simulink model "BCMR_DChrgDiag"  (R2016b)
settings: Solver=FixedStepDiscrete  StartTime=0.0  StopTime=10  FixedStep=0.01  RelTol=1e-3  EnableMultiTasking=on
undefined symbols (not defined in the file or in its folder): BCMR_bDChrgStopCActiveSw_C, BCMR_cntDChrgTCnntMax_C, BCMR_cntIsoFltTrigger_CW, BCMR_EVCCDiagccSw_C, BCMR_EVCCDiagSw_C, BCMR_G1E0PlatformSwDiag_C, BCMR_H1U0PlatformSwDiag_C, BCMR_iDcChrgDiffOvrCurr_C, BCMR_iDcChrgLowTempDiffOvrCurrMody_C, BCMR_iDcChrgLowTempOvrCurrCutOff_C, BCMR_iDcChrgLowTempOvrCurrHeal_C, BCMR_iDcChrgOvrCurr_C, BCMR_iDcChrgOvrVolt_C, BCMR_iDChrgCurrDiagLmt_C, BCMR_iDChrgCutOffVoltOvrCurrDet_C, BCMR_iDChrgCutOffVoltOvrCurrHeal_C, BCMR_kWaveFltFactor_C, BCMR_stCCSTimeout_C, BCMR_stCHMTimeout_C, BCMR_stCMLTimeout_C, BCMR_stCRMAATimeout_C, BCMR_stCROAATimeout_C, BCMR_stCROTimeout_C, BCMR_stCSDTimeout1_C, BCMR_stCSDTimeout2_C, BCMR_stCSTTimeout_C, BCMR_stCurrDwnTimeout_C, BCMR_stHvOnTimeout_C, BCMR_stNoTimeout_C, BCMR_stParaMish_C, BCMR_tBattLowTempDiagTempThrd_C, BCMR_tDcChrgIntfTempDiffLmt_C, BCMR_tDcChrgIntfTempLmt_C, BCMR_tiDChrgDetDiagDebs_C, BCMR_tiDChrgDetSec_C, BCMR_tiDChrgDiagBase_C, BCMR_tiDChrgHealDiagDebs_C, BCMR_tiDChrgIntfTempDwnLmt_C, BCMR_tiDChrgLowTOvrCurrDet_C, BCMR_tiDChrgLowTOvrCurrHeal_C, BCMR_tiDChrgMishCurrDetDiagDebs_C, BCMR_tiDChrgOvrCellVolt_C, BCMR_tiDChrgOvrSafeCellVoltDet_C, BCMR_tiDChrgVoltFltDetDebs_C, BCMR_tiDChrgVoltFltHealDebs_C, BCMR_uCC2ChkDiffDet_C, BCMR_uCC2ChkDiffHeal_C, BCMR_uCC2VoltHighDet_C, BCMR_uCC2VoltHighHeal_C, BCMR_uCC2VoltLowDet_C, BCMR_uCC2VoltLowHeal_C, BCMR_uDChrgHighTempDet_C, BCMR_uDChrgHighTempHeal_C, BCMR_uDChrgLowTempDet_C, BCMR_uDChrgLowTempHeal_C, BCMR_uDChrgOvrCellVoltDet_C, BCMR_uDChrgOvrCellVoltHeal_C, BCMR_uDChrgOvrSafeCellVoltDet_C, BCMR_uDChrgOvrSafeCellVoltHeal_C, bin2dec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
libraries: simulink x291
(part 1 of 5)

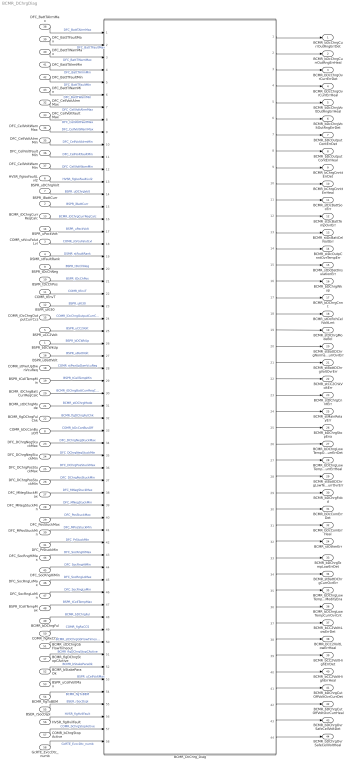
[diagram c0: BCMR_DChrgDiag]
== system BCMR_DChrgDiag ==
  BSPR_bDCWkUp : Inport
  BSPR_iBattCurr : Inport  Port=2
  COMR_stVcuFalutLvl : Inport  Port=3
  DSMR_stFaultRank : Inport  Port=4
  BSPR_uCC2Volt : Inport  Port=5
  HVSR_flgIsoFaultLvl2 : Inport  Port=6
  BSPR_uDChrgVolt : Inport  Port=7
  COMR_bDcCanBusOff : Inport  Port=8
  BSPR_tDcChNeg : Inport  Port=9
  BSPR_tDcChPos : Inport  Port=10
  COMR_tEnvT : Inport  Port=11
  BSPR_uKl30 : Inport  Port=12
  BCMR_iDChrgCurrReqCalc : Inport  Port=13
  BSPR_uPackVolt : Inport  Port=14
  COMR_iDcChrgOutputCurrCcs : Inport  Port=15
  BSPR_uBattVolt : Inport  Port=16
  BCMR_flgDChrgStopCActive : Inport  Port=17
  COMR_stPwrUpDwnVcuReq : Inport  Port=18
  BSPR_tCellTempMin : Inport  Port=19
  BCMR_iDChrgBattCurrReqCalc : Inport  Port=20
  BCMR_stDChrgMode : Inport  Port=21
  BCMR_flgDChrgFulChk : Inport  Port=22
  DFC_DChrgNegStuckMax : Inport  Port=23
  DFC_DChrgNegStuckMin : Inport  Port=24
  DFC_DChrgPosStuckMax : Inport  Port=25
  DFC_DChrgPosStuckMin : Inport  Port=26
  DFC_MNegStuckMax : Inport  Port=27
  DFC_MNegStuckMin : Inport  Port=28
  DFC_PosStuckMax : Inport  Port=29
  DFC_MPosStuckMin : Inport  Port=30
  DFC_PrStuckMin : Inport  Port=31
  DFC_CellVoltAlrmMax : Inport  Port=32
  DFC_CellVoltFaultMax : Inport  Port=33
  DFC_CellVoltWarnMax : Inport  Port=34
  DFC_CellVoltAlrmMin : Inport  Port=35
  DFC_CellVoltFaultMin : Inport  Port=36
  DFC_CellVoltWarnMin : Inport  Port=37
  DFC_BattTAlrmMax : Inport  Port=38
  DFC_BattTFaultMax : Inport  Port=39
  "DFC_BattTWarnMax " : Inport  Port=40
  DFC_BattTAlrmMin : Inport  Port=41
  DFC_BattTFaultMin : Inport  Port=42
  DFC_BattTWarnMin : Inport  Port=43
  DFC_SocRngHiMax : Inport  Port=44
  DFC_SocRngHiMin : Inport  Port=45
  DFC_SocRngLoMax : Inport  Port=46
  DFC_SocRngLoMin : Inport  Port=47
  BSPR_tCellTempMax : Inport  Port=48
  BCMR_bDChrgFul : Inport  Port=49
  COMR_flgRxCCS : Inport  Port=50
  BCMR_stDChrgGbFlowTimeout : Inport  Port=51
  BCMR_bStakeParaOk : Inport  Port=52
  BSPR_uCellVoltMax : Inport  Port=53
  BCMR_flgTxBEM : Inport  Port=54
  BSER_rSocDspl : Inport  Port=55
  HVSR_flgHvilFault : Inport  Port=56
  COMR_bChrgStopActive : Inport  Port=57
  GcRTE_EvccDtc_numb : Inport  Port=58
  BCMR_DcChrg_Diag : Subsystem
  BCMR_bDcChrgCurrOutRngErrDet : Outport  InitialOutput=[0]
  BCMR_bDcChrgCurrOutRngErrHeal : Outport  Port=2  InitialOutput=[0]
  BCMR_bDcChrgOvrCurrErrDet : Outport  Port=3  InitialOutput=[0]
  BCMR_bDcChrgOvrCurrErrHeal : Outport  Port=4  InitialOutput=[0]
  BCMR_bDcChrgVoltOutRngErrHeal : Outport  Port=5  InitialOutput=[0]
  BCMR_bDcChrgVoltOutRngErrDet : Outport  Port=6  InitialOutput=[0]
  BCMR_bDcOutputContErrDet : Outport  Port=7  InitialOutput=[0]
  BCMR_bDcOutputContErrHeal : Outport  Port=8  InitialOutput=[0]
  BCMR_bChrgCnnttErrDet : Outport  Port=9  InitialOutput=[0]
  BCMR_bChrgCnnttErrHeal : Outport  Port=10  InitialOutput=[0]
  BCMR_stDcBattSocErr : Outport  Port=11
  BCMR_stDcBattTempOvrErr : Outport  Port=12
  BCMR_stDcBattCellVoltErr : Outport  Port=13
  BCMR_stDcOutpCnntOvrTempErr : Outport  Port=14  OutDataTypeStr=uint8
  BCMR_stDcBattInsulationErr : Outport  Port=15
  BCMR_bDChrgWkup : Outport  Port=16
  BCMR_bDChrgCnnt : Outport  Port=17
  BCMR_stDcRchCellVoltLmt : Outport  Port=18  OutDataTypeStr=uint8
  BCMR_stDChrgModeBcl : Outport  Port=19  InitialOutput=[0]
  BCMR_stBattDChrgNormalTempCurrOvrErr : Outport  Port=20
  BCMR_stBattDChrgVoltOvrErr : Outport  Port=21
  BCMR_stCC2ChkVoltErr : Outport  Port=22
  BCMR_stDChrgCnntErr : Outport  Port=23  InitialOutput=[0]
  BCMR_stOtherErr : Outport  Port=24
  BCMR_stMainRelayErr : Outport  Port=25
  BCMR_bDChrgStopEna : Outport  Port=26
  BCMR_bDChrgLowTempOvrCurrErrDet : Outport  Port=27
  BCMR_bDChrgLowTempOvrCurrErrHeal : Outport  Port=28
  BCMR_stBattDChrgLowTempCurrOvrErr : Outport  Port=29
  BCMR_bDChrgFobd : Outport  Port=30
  BCMR_bDcComErrDet : Outport  Port=31
  BCMR_bDcComErrHeal : Outport  Port=32
  BCMR_bDChrgTempLowErrDet : Outport  Port=33
  BCMR_stBattDChrgCurrOvrErr : Outport  Port=34  InitialOutput=[0]
  BCMR_bDChrgLowTempCurrModifyEna : Outport  Port=35
  BCMR_bDChrgLowTempCurrOvrCnt : Outport  Port=36  OutputWhenDisabled=reset  InitialOutput=[0]
  BCMR_bCC2VolttLowErrDet : Outport  Port=37  InitialOutput=[0]
  BCMR_bCC2VoltLowErrHeal : Outport  Port=38  InitialOutput=[0]
  BCMR_bCC2VoltHighErrDet : Outport  Port=39  InitialOutput=[0]
  BCMR_bCC2VoltHighErrHeal : Outport  Port=40  InitialOutput=[0]
  BCMR_bDChrgCutOffVoltOvrCurrDet : Outport  Port=41
  BCMR_bDChrgCutOffVoltOvrCurrHeal : Outport  Port=42
  BCMR_bDChrgOvrSafeCellVoltDet : Outport  Port=43
  BCMR_bDChrgOvrSafeCellVoltHeal : Outport  Port=44
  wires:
  HVSR_flgIsoFaultLvl2/1 -> BCMR_DcChrg_Diag/13(HVSR_flgIsoFaultLvl2)  "HVSR_flgIsoFaultLvl2"
  BSPR_uDChrgVolt/1 -> BCMR_DcChrg_Diag/14(BSPR_uDChrgVolt)  "BSPR_uDChrgVolt"
  BSPR_iBattCurr/1 -> BCMR_DcChrg_Diag/15(BSPR_iBattCurr)  "BSPR_iBattCurr"
  COMR_bDcCanBusOff/1 -> BCMR_DcChrg_Diag/33(COMR_bDcCanBusOff)  "COMR_bDcCanBusOff"
  COMR_stVcuFalutLvl/1 -> BCMR_DcChrg_Diag/18(COMR_stVcuFalutLvl)  "COMR_stVcuFalutLvl"
  DSMR_stFaultRank/1 -> BCMR_DcChrg_Diag/19(DSMR_stFaultRank)  "DSMR_stFaultRank"
  BSPR_tDcChNeg/1 -> BCMR_DcChrg_Diag/20(BSPR_tDcChNeg)  "BSPR_tDcChNeg"
  BSPR_tDcChPos/1 -> BCMR_DcChrg_Diag/21(BSPR_tDcChPos)  "BSPR_tDcChPos"
  BSPR_uKl30/1 -> BCMR_DcChrg_Diag/23(BSPR_uKl30)  "BSPR_uKl30"
  COMR_tEnvT/1 -> BCMR_DcChrg_Diag/22(COMR_tEnvT)  "COMR_tEnvT"
  BSPR_bDCWkUp/1 -> BCMR_DcChrg_Diag/26(BSPR_bDCWkUp)  "BSPR_bDCWkUp"
  BSPR_uCC2Volt/1 -> BCMR_DcChrg_Diag/25(BSPR_uCC2Volt)  "BSPR_uCC2Volt"
  BCMR_iDChrgCurrReqCalc/1 -> BCMR_DcChrg_Diag/16(BCMR_iDChrgCurrReqCalc)  "BCMR_iDChrgCurrReqCalc"
  BSPR_uPackVolt/1 -> BCMR_DcChrg_Diag/17(BSPR_uPackVolt)  "BSPR_uPackVolt"
  COMR_iDcChrgOutputCurrCcs/1 -> BCMR_DcChrg_Diag/24(COMR_iDcChrgOutputCurrCcs)  "COMR_iDcChrgOutputCurrCcs"
  BSPR_uBattVolt/1 -> BCMR_DcChrg_Diag/27(BSPR_uBattVolt)  "BSPR_uBattVolt"
  BCMR_flgDChrgStopCActive/1 -> BCMR_DcChrg_Diag/51(BCMR_flgDChrgStopCActive)  "BCMR_flgDChrgStopCActive"
  BCMR_DcChrg_Diag/13(BCMR_stDcBattCellVoltErr) -> BCMR_stDcBattCellVoltErr/1
  BCMR_DcChrg_Diag/22(BCMR_stCC2ChkVoltErr) -> BCMR_stCC2ChkVoltErr/1
  BCMR_DcChrg_Diag/1(BCMR_bDcChrgCurrOutRngErrDet) -> BCMR_bDcChrgCurrOutRngErrDet/1
  BCMR_DcChrg_Diag/2(BCMR_bDcChrgCurrOutRngErrHeal) -> BCMR_bDcChrgCurrOutRngErrHeal/1
  BCMR_DcChrg_Diag/3(BCMR_bDcChrgOvrCurrErrDet) -> BCMR_bDcChrgOvrCurrErrDet/1
  BCMR_DcChrg_Diag/4(BCMR_bDcChrgOvrCurrErrHeal) -> BCMR_bDcChrgOvrCurrErrHeal/1
  BCMR_DcChrg_Diag/6(BCMR_bDcChrgVoltOutRngErrDet) -> BCMR_bDcChrgVoltOutRngErrDet/1
  BCMR_DcChrg_Diag/5(BCMR_bDcChrgVoltOutRngErrHeal) -> BCMR_bDcChrgVoltOutRngErrHeal/1
  BCMR_DcChrg_Diag/7(BCMR_bDcOutputContErrDet) -> BCMR_bDcOutputContErrDet/1
  BCMR_DcChrg_Diag/8(BCMR_bDcOutputContErrHeal) -> BCMR_bDcOutputContErrHeal/1
  BCMR_DcChrg_Diag/9(BCMR_bChrgCnnttErrDet) -> BCMR_bChrgCnnttErrDet/1
  BCMR_DcChrg_Diag/10(BCMR_bChrgCnnttErrHeal) -> BCMR_bChrgCnnttErrHeal/1
  BCMR_DcChrg_Diag/11(BCMR_stDcBattSocErr) -> BCMR_stDcBattSocErr/1
  BCMR_DcChrg_Diag/12(BCMR_stDcBattTempOvrErr) -> BCMR_stDcBattTempOvrErr/1
  BCMR_DcChrg_Diag/16(BCMR_bDChrgWkup) -> BCMR_bDChrgWkup/1
  BCMR_DcChrg_Diag/17(BCMR_bDChrgCnnt) -> BCMR_bDChrgCnnt/1
  BCMR_DcChrg_Diag/18(BCMR_stDcRchCellVoltLmt) -> BCMR_stDcRchCellVoltLmt/1
  BCMR_DcChrg_Diag/15(BCMR_stDcBattInsulationErr) -> BCMR_stDcBattInsulationErr/1
  BCMR_DcChrg_Diag/14(BCMR_stDcOutpCnntOvrTempErr) -> BCMR_stDcOutpCnntOvrTempErr/1
  BCMR_DcChrg_Diag/19(BCMR_stDChrgModeBcl) -> BCMR_stDChrgModeBcl/1
  BCMR_DcChrg_Diag/20(BCMR_stBattNormalTempDChrgCurrOvrErr) -> BCMR_stBattDChrgNormalTempCurrOvrErr/1
  BCMR_DcChrg_Diag/23(BCMR_stDChrgCnntErr) -> BCMR_stDChrgCnntErr/1
  BCMR_DcChrg_Diag/21(BCMR_stBattDChrgVoltOvrErr) -> BCMR_stBattDChrgVoltOvrErr/1
  BCMR_DcChrg_Diag/32(BCMR_stOtherErr) -> BCMR_stOtherErr/1
  BCMR_DcChrg_Diag/24(BCMR_stMainRelayErr) -> BCMR_stMainRelayErr/1
  COMR_stPwrUpDwnVcuReq/1 -> BCMR_DcChrg_Diag/28(COMR_stPwrUpDwnVcuReq)  "COMR_stPwrUpDwnVcuReq"
  BCMR_DcChrg_Diag/25(BCMR_bDChrgStopEna) -> BCMR_bDChrgStopEna/1
  BSPR_tCellTempMin/1 -> BCMR_DcChrg_Diag/29(BSPR_tBattTempMin)  "BSPR_tCellTempMin"
  BCMR_iDChrgBattCurrReqCalc/1 -> BCMR_DcChrg_Diag/30(BCMR_iDChrgBattCurrReqCalc)  "BCMR_iDChrgBattCurrReqCalc"
  BCMR_DcChrg_Diag/26(BCMR_bDChrgLowTempOvrCurrErrDet) -> BCMR_bDChrgLowTempOvrCurrErrDet/1
  BCMR_DcChrg_Diag/27(BCMR_bDChrgLowTempOvrCurrErrHeal) -> BCMR_bDChrgLowTempOvrCurrErrHeal/1
  BCMR_DcChrg_Diag/28(BCMR_stBattDChrgLowTempCurrOvrErr) -> BCMR_stBattDChrgLowTempCurrOvrErr/1
  BCMR_DcChrg_Diag/29(BCMR_bDChrgFobd) -> BCMR_bDChrgFobd/1
  BCMR_stDChrgMode/1 -> BCMR_DcChrg_Diag/31(BCMR_stDChrgMode)  "BCMR_stDChrgMode"
  BCMR_flgDChrgFulChk/1 -> BCMR_DcChrg_Diag/32(BCMR_flgDChrgFulChk)  "BCMR_flgDChrgFulChk"
  BCMR_DcChrg_Diag/31(BCMR_bDcComErrHeal) -> BCMR_bDcComErrHeal/1
  BCMR_DcChrg_Diag/30(BCMR_bDcComErrDet) -> BCMR_bDcComErrDet/1
  DFC_DChrgNegStuckMax/1 -> BCMR_DcChrg_Diag/34(DFC_DChrgNegStuckMax)  "DFC_DChrgNegStuckMax"
  DFC_DChrgNegStuckMin/1 -> BCMR_DcChrg_Diag/35(DFC_DChrgNegStuckMin)  "DFC_DChrgNegStuckMin"
  DFC_DChrgPosStuckMax/1 -> BCMR_DcChrg_Diag/36(DFC_DChrgPosStuckMax)  "DFC_DChrgPosStuckMax"
  DFC_DChrgPosStuckMin/1 -> BCMR_DcChrg_Diag/37(DFC_DChrgPosStuckMin)  "DFC_DChrgPosStuckMin"
  DFC_MNegStuckMax/1 -> BCMR_DcChrg_Diag/38(DFC_MNegStuckMax)  "DFC_MNegStuckMax"
  DFC_MNegStuckMin/1 -> BCMR_DcChrg_Diag/39(DFC_MNegStuckMin)  "DFC_MNegStuckMin"
  DFC_PosStuckMax/1 -> BCMR_DcChrg_Diag/40(DFC_PosStuckMax)  "DFC_PosStuckMax"
  DFC_MPosStuckMin/1 -> BCMR_DcChrg_Diag/41(DFC_MPosStuckMin)  "DFC_MPosStuckMin"
  DFC_PrStuckMin/1 -> BCMR_DcChrg_Diag/42(DFC_PrStuckMin)  "DFC_PrStuckMin"
  DFC_CellVoltAlrmMax/1 -> BCMR_DcChrg_Diag/7(DFC_CellVoltAlrmMax)  "DFC_CellVoltAlrmMax"
  DFC_CellVoltFaultMin/1 -> BCMR_DcChrg_Diag/11(DFC_CellVoltFaultMin)  "DFC_CellVoltFaultMin"
  DFC_CellVoltFaultMax/1 -> BCMR_DcChrg_Diag/8(DFC_CellVoltFaultMax)  "DFC_CellVoltFaultMax"
  DFC_CellVoltWarnMax/1 -> BCMR_DcChrg_Diag/9(DFC_CellVoltWarnMax)  "DFC_CellVoltWarnMax"
  DFC_CellVoltAlrmMin/1 -> BCMR_DcChrg_Diag/10(DFC_CellVoltAlrmMin)  "DFC_CellVoltAlrmMin"
  DFC_CellVoltWarnMin/1 -> BCMR_DcChrg_Diag/12(DFC_CellVoltWarnMin)  "DFC_CellVoltWarnMin"
  DFC_BattTAlrmMax/1 -> BCMR_DcChrg_Diag/1(DFC_BattTAlrmMax)  "DFC_BattTAlrmMax"
  DFC_BattTFaultMax/1 -> BCMR_DcChrg_Diag/2(DFC_BattTFaultMax)  "DFC_BattTFaultMax"
  "DFC_BattTWarnMax "/1 -> BCMR_DcChrg_Diag/3("DFC_BattTWarnMax ")  "DFC_BattTWarnMax"
  DFC_BattTAlrmMin/1 -> BCMR_DcChrg_Diag/4(DFC_BattTAlrmMin)  "DFC_BattTAlrmMin"
  DFC_BattTFaultMin/1 -> BCMR_DcChrg_Diag/5(DFC_BattTFaultMin)  "DFC_BattTFaultMin"
  DFC_BattTWarnMin/1 -> BCMR_DcChrg_Diag/6(DFC_BattTWarnMin)  "DFC_BattTWarnMin"
  DFC_SocRngHiMax/1 -> BCMR_DcChrg_Diag/43(DFC_SocRngHiMax)  "DFC_SocRngHiMax"
  DFC_SocRngHiMin/1 -> BCMR_DcChrg_Diag/44(DFC_SocRngHiMin)  "DFC_SocRngHiMin"
  DFC_SocRngLoMax/1 -> BCMR_DcChrg_Diag/45(DFC_SocRngLoMax)  "DFC_SocRngLoMax"
  DFC_SocRngLoMin/1 -> BCMR_DcChrg_Diag/46(DFC_SocRngLoMin)  "DFC_SocRngLoMin"
  BCMR_DcChrg_Diag/33(BCMR_bDChrgTempLowErrDet) -> BCMR_bDChrgTempLowErrDet/1
  BSPR_tCellTempMax/1 -> BCMR_DcChrg_Diag/47(BSPR_tBattTempMax)  "BSPR_tCellTempMax"
  BCMR_DcChrg_Diag/34(BCMR_stBattDChrgCurrOvrErr) -> BCMR_stBattDChrgCurrOvrErr/1
  BCMR_bDChrgFul/1 -> BCMR_DcChrg_Diag/48(BCMR_bDChrgFul)  "BCMR_bDChrgFul"
  COMR_flgRxCCS/1 -> BCMR_DcChrg_Diag/49(COMR_flgRxCCS)  "COMR_flgRxCCS"
  BCMR_DcChrg_Diag/35(BCMR_bDChrgLowTempCurrModifyEna) -> BCMR_bDChrgLowTempCurrModifyEna/1
  BCMR_DcChrg_Diag/36(BCMR_bDChrgLowTempCurrOvrCnt) -> BCMR_bDChrgLowTempCurrOvrCnt/1
  BCMR_stDChrgGbFlowTimeout/1 -> BCMR_DcChrg_Diag/50(BCMR_stDChrgGbFlowTimeout)  "BCMR_stDChrgGbFlowTimeout"
  BCMR_bStakeParaOk/1 -> BCMR_DcChrg_Diag/52(BCMR_bStakeParaOk)  "BCMR_bStakeParaOk"
  BCMR_DcChrg_Diag/37(BCMR_bCC2VolttLowErrDet) -> BCMR_bCC2VolttLowErrDet/1
  BCMR_DcChrg_Diag/40(BCMR_bCC2VoltHighErrHeal) -> BCMR_bCC2VoltHighErrHeal/1
  BCMR_DcChrg_Diag/39(BCMR_bCC2VoltHighErrDet) -> BCMR_bCC2VoltHighErrDet/1
  BCMR_DcChrg_Diag/38(BCMR_bCC2VoltLowErrHeal) -> BCMR_bCC2VoltLowErrHeal/1
  BCMR_DcChrg_Diag/41(BCMR_bDChrgCutOffVoltOvrCurrDet) -> BCMR_bDChrgCutOffVoltOvrCurrDet/1
  BCMR_DcChrg_Diag/42(BCMR_bDChrgCutOffVoltOvrCurrHeal) -> BCMR_bDChrgCutOffVoltOvrCurrHeal/1
  BSPR_uCellVoltMax/1 -> BCMR_DcChrg_Diag/53(BSPR_uCellVoltMax)  "BSPR_uCellVoltMax"
  BCMR_flgTxBEM/1 -> BCMR_DcChrg_Diag/54(BCMR_flgTxBEM)  "BCMR_flgTxBEM"
  BSER_rSocDspl/1 -> BCMR_DcChrg_Diag/55(BSER_rSocDspl)  "BSER_rSocDspl"
  HVSR_flgHvilFault/1 -> BCMR_DcChrg_Diag/56(HVSR_flgHvilFault)  "HVSR_flgHvilFault"
  BCMR_DcChrg_Diag/43(BCMR_bDChrgOvrSafeCellVoltDet) -> BCMR_bDChrgOvrSafeCellVoltDet/1
  BCMR_DcChrg_Diag/44(BCMR_bDChrgOvrSafeCellVoltHeal) -> BCMR_bDChrgOvrSafeCellVoltHeal/1
  COMR_bChrgStopActive/1 -> BCMR_DcChrg_Diag/57(COMR_bChrgStopActive)  "COMR_bChrgStopActive"
  GcRTE_EvccDtc_numb/1 -> BCMR_DcChrg_Diag/58(GcRTE_EvccDtc_numb)  "GcRTE_EvccDtc_numb"

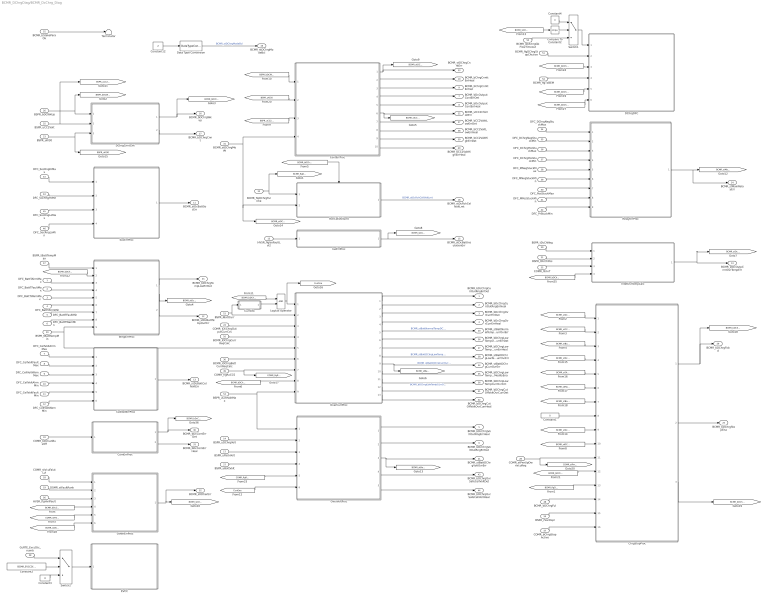
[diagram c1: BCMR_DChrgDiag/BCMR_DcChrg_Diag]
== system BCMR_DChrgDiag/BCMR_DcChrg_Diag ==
  DFC_BattTAlrmMax : Inport
  DFC_BattTFaultMax : Inport  Port=2
  "DFC_BattTWarnMax " : Inport  Port=3
  DFC_BattTAlrmMin : Inport  Port=4
  DFC_BattTFaultMin : Inport  Port=5
  DFC_BattTWarnMin : Inport  Port=6
  DFC_CellVoltAlrmMax : Inport  Port=7
  DFC_CellVoltFaultMax : Inport  Port=8
  DFC_CellVoltWarnMax : Inport  Port=9
  DFC_CellVoltAlrmMin : Inport  Port=10
  DFC_CellVoltFaultMin : Inport  Port=11
  DFC_CellVoltWarnMin : Inport  Port=12
  HVSR_flgIsoFaultLvl2 : Inport  Port=13
  BSPR_uDChrgVolt : Inport  Port=14
  BSPR_iBattCurr : Inport  Port=15
  BCMR_iDChrgCurrReqCalc : Inport  Port=16
  BSPR_uPackVolt : Inport  Port=17
  COMR_stVcuFalutLvl : Inport  Port=18
  DSMR_stFaultRank : Inport  Port=19
  BSPR_tDcChNeg : Inport  Port=20
  BSPR_tDcChPos : Inport  Port=21
  COMR_tEnvT : Inport  Port=22
  BSPR_uKl30 : Inport  Port=23
  COMR_iDcChrgOutputCurrCcs : Inport  Port=24
  BSPR_uCC2Volt : Inport  Port=25
  BSPR_bDCWkUp : Inport  Port=26
  BSPR_uBattVolt : Inport  Port=27
  COMR_stPwrUpDwnVcuReq : Inport  Port=28
  BSPR_tBattTempMin : Inport  Port=29
  BCMR_iDChrgBattCurrReqCalc : Inport  Port=30
  BCMR_stDChrgMode : Inport  Port=31
  BCMR_flgDChrgFulChk : Inport  Port=32
  COMR_bDcCanBusOff : Inport  Port=33
  DFC_DChrgNegStuckMax : Inport  Port=34
  DFC_DChrgNegStuckMin : Inport  Port=35
  DFC_DChrgPosStuckMax : Inport  Port=36
  DFC_DChrgPosStuckMin : Inport  Port=37
  DFC_MNegStuckMax : Inport  Port=38
  DFC_MNegStuckMin : Inport  Port=39
  DFC_PosStuckMax : Inport  Port=40
  DFC_MPosStuckMin : Inport  Port=41
  DFC_PrStuckMin : Inport  Port=42
  DFC_SocRngHiMax : Inport  Port=43
  DFC_SocRngHiMin : Inport  Port=44
  DFC_SocRngLoMax : Inport  Port=45
  DFC_SocRngLoMin : Inport  Port=46
  BSPR_tBattTempMax : Inport  Port=47
  BCMR_bDChrgFul : Inport  Port=48
  COMR_flgRxCCS : Inport  Port=49
  BCMR_stDChrgGbFlowTimeout : Inport  Port=50
  BCMR_flgDChrgStopCActive : Inport  Port=51
  BCMR_bStakeParaOk : Inport  Port=52
  BSPR_uCellVoltMax : Inport  Port=53
  BCMR_flgTxBEM : Inport  Port=54
  BSER_rSocDspl : Inport  Port=55
  HVSR_flgHvilFault : Inport  Port=56
  COMR_bChrgStopActive : Inport  Port=57
  GcRTE_EvccDtc_numb : Inport  Port=58
  CellVoltErrProc : Subsystem  TreatAsAtomicUnit=on
  ChrgStopProc : Subsystem  TreatAsAtomicUnit=on
  ComErrProc : Subsystem  TreatAsAtomicUnit=on
  Compare To Constant2 : simulink/Logic and Bit Operations/Compare To Constant  relop===  const=1  OutDataTypeStr=boolean
  Constant1 : Constant  Value=0  OutDataTypeStr=uint8
  Constant12 : Constant  Value=2  OutDataTypeStr=uint8  SampleTime=-1
  Constant2 : Constant  Value=BCMR_EVCCDiagSw_C
  Constant3 : Constant  Value=0
  Constant4 : Constant  Value=0  OutDataTypeStr=single
  ContErrProc : Subsystem  TreatAsAtomicUnit=on
  CurrChk : Subsystem
  DChrgCnntChk : Subsystem  TreatAsAtomicUnit=on
  DChrgDFC : Subsystem  TreatAsAtomicUnit=on
  Data Type Conversion : DataTypeConversion  OutDataTypeStr=uint8
  EVCC : Subsystem
  IntetOvrTempCalc : Subsystem  TreatAsAtomicUnit=on
  IsoErrProc : Subsystem  TreatAsAtomicUnit=on
  Logical Operator : Logic  AllPortsSameDT=off  OutDataTypeStr=boolean
  OtherErrProc : Subsystem  TreatAsAtomicUnit=on
  OverCurrProc : Subsystem  TreatAsAtomicUnit=on
  OverVoltProc : Subsystem  TreatAsAtomicUnit=on
  RchCellVoltLmt : Subsystem  TreatAsAtomicUnit=on
  RelayErrProc : Subsystem  TreatAsAtomicUnit=on
  SocErrProc : Subsystem  TreatAsAtomicUnit=on
  Switch1 : Switch  Criteria=u2 ~= 0
  Switch2 : Switch  Criteria=u2 ~= 0
  TempErrProc : Subsystem  TreatAsAtomicUnit=on
  Terminator : Terminator
  BCMR_bDcChrgCurrOutRngErrDet : Outport  InitialOutput=[0]
  BCMR_bDcChrgCurrOutRngErrHeal : Outport  Port=2  InitialOutput=[0]
  BCMR_bDcChrgOvrCurrErrDet : Outport  Port=3  InitialOutput=[0]
  BCMR_bDcChrgOvrCurrErrHeal : Outport  Port=4  InitialOutput=[0]
  BCMR_bDcChrgVoltOutRngErrHeal : Outport  Port=5  InitialOutput=[0]
  BCMR_bDcChrgVoltOutRngErrDet : Outport  Port=6  InitialOutput=[0]
  BCMR_bDcOutputContErrDet : Outport  Port=7  InitialOutput=[0]
  BCMR_bDcOutputContErrHeal : Outport  Port=8  InitialOutput=[0]
  BCMR_bChrgCnnttErrDet : Outport  Port=9  InitialOutput=[0]
  BCMR_bChrgCnnttErrHeal : Outport  Port=10  InitialOutput=[0]
  BCMR_stDcBattSocErr : Outport  Port=11
  BCMR_stDcBattTempOvrErr : Outport  Port=12
  BCMR_stDcBattCellVoltErr : Outport  Port=13
  BCMR_stDcOutpCnntOvrTempErr : Outport  Port=14  OutDataTypeStr=uint8
  BCMR_stDcBattInsulationErr : Outport  Port=15
  BCMR_bDChrgWkup : Outport  Port=16
  BCMR_bDChrgCnnt : Outport  Port=17
  BCMR_stDcRchCellVoltLmt : Outport  Port=18  OutDataTypeStr=uint8
  BCMR_stDChrgModeBcl : Outport  Port=19  InitialOutput=[0]
  BCMR_stBattNormalTempDChrgCurrOvrErr : Outport  Port=20
  BCMR_stBattDChrgVoltOvrErr : Outport  Port=21
  BCMR_stCC2ChkVoltErr : Outport  Port=22
  BCMR_stDChrgCnntErr : Outport  Port=23  InitialOutput=[0]
  BCMR_stMainRelayErr : Outport  Port=24
  BCMR_bDChrgStopEna : Outport  Port=25
  BCMR_bDChrgLowTempOvrCurrErrDet : Outport  Port=26
  BCMR_bDChrgLowTempOvrCurrErrHeal : Outport  Port=27
  BCMR_stBattDChrgLowTempCurrOvrErr : Outport  Port=28
  BCMR_bDChrgFobd : Outport  Port=29
  BCMR_bDcComErrDet : Outport  Port=30
  BCMR_bDcComErrHeal : Outport  Port=31
  BCMR_stOtherErr : Outport  Port=32
  BCMR_bDChrgTempLowErrDet : Outport  Port=33
  BCMR_stBattDChrgCurrOvrErr : Outport  Port=34  InitialOutput=[0]
  BCMR_bDChrgLowTempCurrModifyEna : Outport  Port=35
  BCMR_bDChrgLowTempCurrOvrCnt : Outport  Port=36  OutputWhenDisabled=reset  InitialOutput=[0]
  BCMR_bCC2VolttLowErrDet : Outport  Port=37  InitialOutput=[0]
  BCMR_bCC2VoltLowErrHeal : Outport  Port=38  InitialOutput=[0]
  BCMR_bCC2VoltHighErrDet : Outport  Port=39  InitialOutput=[0]
  BCMR_bCC2VoltHighErrHeal : Outport  Port=40  InitialOutput=[0]
  BCMR_bDChrgCutOffVoltOvrCurrDet : Outport  Port=41
  BCMR_bDChrgCutOffVoltOvrCurrHeal : Outport  Port=42
  BCMR_bDChrgOvrSafeCellVoltDet : Outport  Port=43
  BCMR_bDChrgOvrSafeCellVoltHeal : Outport  Port=44
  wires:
  SocErrProc/1(BCMR_stDcBattSocErr) -> BCMR_stDcBattSocErr/1
  DFC_CellVoltAlrmMax/1 -> CellVoltErrProc/1(DFC_CellVoltAlrmMax)
  DFC_CellVoltFaultMax/1 -> CellVoltErrProc/2(DFC_CellVoltFaultMax)
  DFC_CellVoltWarnMax/1 -> CellVoltErrProc/3(DFC_CellVoltWarnMax)
  DFC_CellVoltAlrmMin/1 -> CellVoltErrProc/4(DFC_CellVoltAlrmMin)
  DFC_CellVoltFaultMin/1 -> CellVoltErrProc/5(DFC_CellVoltFaultMin)
  DFC_CellVoltWarnMin/1 -> CellVoltErrProc/6(DFC_CellVoltWarnMin)
  CellVoltErrProc/1(BCMR_stDcBattCellVoltErr) -> BCMR_stDcBattCellVoltErr/1
  HVSR_flgIsoFaultLvl2/1 -> IsoErrProc/1(HVSR_flgIsoFaultLvl2)
  IsoErrProc/1(BCMR_stDcBattInsulationErr) -> [BCMR_stDcBattInsulationErr], BCMR_stDcBattInsulationErr/1
  BCMR_iDChrgCurrReqCalc/1 -> OverCurrProc/4(BCMR_iDChrgCurrReqCalc)
  OverCurrProc/1(BCMR_bDcChrgCurrOutRngErrDet) -> BCMR_bDcChrgCurrOutRngErrDet/1
  OverCurrProc/2(BCMR_bDcChrgCurrOutRngErrHeal) -> BCMR_bDcChrgCurrOutRngErrHeal/1
  OverCurrProc/3(BCMR_bDcChrgOvrCurrErrDet) -> BCMR_bDcChrgOvrCurrErrDet/1
  OverCurrProc/4(BCMR_bDcChrgOvrCurrErrHeal) -> BCMR_bDcChrgOvrCurrErrHeal/1
  OverCurrProc/5(BCMR_stBattNormalTempDChrgCurrOvrErr) -> BCMR_stBattNormalTempDChrgCurrOvrErr/1  "BCMR_stBattNormalTempDChrgCurrOvrErr"
  BSPR_uPackVolt/1 -> OverVoltProc/3(BSPR_uPackVolt)
  Constant12/1 -> Data Type Conversion/1
  RelayErrProc/1(BCMR_stMainRelayErr) -> BCMR_stMainRelayErr/1, [BCMR_stMainRelayErr]
  BSPR_iBattCurr/1 -> CurrChk/1(Curr), OverCurrProc/2(BSPR_iBattCurr)
  OverVoltProc/1(BCMR_bDcChrgVoltOutRngErrHeal) -> BCMR_bDcChrgVoltOutRngErrHeal/1
  OverVoltProc/2(BCMR_bDcChrgVoltOutRngErrDet) -> BCMR_bDcChrgVoltOutRngErrDet/1
  OverVoltProc/3(BCMR_stBattDChrgVoltOvrErr) -> [BCMR_stBattDChrgVoltOvrErr], BCMR_stBattDChrgVoltOvrErr/1
  BSPR_uBattVolt/1 -> OverVoltProc/4(BSPR_uBattVolt)
  COMR_iDcChrgOutputCurrCcs/1 -> OverCurrProc/3(COMR_iDcChrgOutputCurrCcs)
  TempErrProc/2(BCMR_stDcBattTempOvrErr) -> [BCMR_stDcBattTempOvrErr], BCMR_stDcBattTempOvrErr/1
  BSPR_tDcChPos/1 -> IntetOvrTempCalc/2(BSPR_tDcChPos)
  COMR_tEnvT/1 -> IntetOvrTempCalc/3(COMR_tEnvT)
  BSPR_tDcChNeg/1 -> IntetOvrTempCalc/1(BSPR_tDcChNeg)
  IntetOvrTempCalc/1(BCMR_stDcOutpCnntOvrTempErr) -> [BCMR_stDcOutpCnntOvrTempErr], BCMR_stDcOutpCnntOvrTempErr/1
  BSPR_uCC2Volt/1 -> DChrgCnntChk/2(BSPR_uCC2Volt), [BSPR_uCC2Volt]
  BSPR_bDCWkUp/1 -> DChrgCnntChk/1(BSPR_bDCWkUp), [BSPR_bDCWkUp]
  [BCMR_bDChrgWkup] -> RchCellVoltLmt/Enable
  RchCellVoltLmt/1(BCMR_stDcRchCellVoltLmt) -> BCMR_stDcRchCellVoltLmt/1  "BCMR_stDcRchCellVoltLmt"
  BCMR_flgDChrgFulChk/1 -> RchCellVoltLmt/1(BCMR_flgDChrgFulChk), [BCMR_flgDChgFulChk]
  [BSPR_uCC2Volt] -> ContErrProc/3(BSPR_uCC2Volt)
  [BSPR_bDCWkUp] -> ContErrProc/1(BSPR_bDCWkUp)
  [BCMR_bDChrgWkup] -> Logical Operator/1
  [BCMR_flgDChgFulChk] -> ChrgStopProc/13(BCMR_flgDChgFulChk)
  [BCMR_stDcBattTempOvrErr] -> ChrgStopProc/1(BCMR_stDcBattTempOvrErr)
  [BCMR_stCC2ChkVoltErr] -> ChrgStopProc/2(BCMR_stCC2ChkVoltErr)
  [BCMR_stBattDChrgCurrOvrErr] -> ChrgStopProc/3(BCMR_stBattDChrgCurrOvrErr)
  [BCMR_stDcOutpCnntOvrTempErr] -> ChrgStopProc/9(BCMR_stDcOutpCnntOvrTempErr)
  [BCMR_stDcBattInsulationErr] -> ChrgStopProc/4(BCMR_stDcBattInsulationErr)
  [BCMR_stOtherErr] -> ChrgStopProc/5(BCMR_stOtherErr)
  [BCMR_stMainRelayErr] -> ChrgStopProc/6(BCMR_stMainRelayErr)
  [BCMR_stBattDChrgVoltOvrErr] -> ChrgStopProc/7(BCMR_stBattDChrgVoltOvrErr)
  Constant1/1 -> ChrgStopProc/8(BCMR_stPcbOvrTempErr)
  COMR_stPwrUpDwnVcuReq/1 -> [COMR_stPwrUpDwnVcuReq], ChrgStopProc/11(COMR_stPwrUpDwnVcuReq)
  BSPR_tBattTempMin/1 -> TempErrProc/9(BSPR_tBattTempMin), OverCurrProc/5(BSPR_tBattTempMin)
  BCMR_iDChrgBattCurrReqCalc/1 -> OverCurrProc/6(BCMR_iDChrgBattCurrReqCalc)
  OverCurrProc/6(BCMR_bDChrgLowTempOvrCurrErrDet) -> BCMR_bDChrgLowTempOvrCurrErrDet/1
  OverCurrProc/7(BCMR_bDChrgLowTempOvrCurrErrHeal) -> BCMR_bDChrgLowTempOvrCurrErrHeal/1
  OverCurrProc/8(BCMR_stBattDChrgLowTempCurrOvrErr) -> BCMR_stBattDChrgLowTempCurrOvrErr/1  "BCMR_stBattDChrgLowTempCurrOvrErr"
  BCMR_stDChrgMode/1 -> ContErrProc/4(BCMR_stDChrgMode), [BCMR_stDChrgMode], RchCellVoltLmt/2(BCMR_stDChrgMode)
  ChrgStopProc/2(BCMR_bDChrgStopEna) -> BCMR_bDChrgStopEna/1
  ChrgStopProc/1(BCMR_bDChrgFobd) -> [BCMR_bDChrgFobd], BCMR_bDChrgFobd/1
  [BCMR_bDChrgWkup] -> ChrgStopProc/12(BCMR_bDChrgWkup)
  COMR_bDcCanBusOff/1 -> ComErrProc/1(COMR_bDcCanBusOff)
  ComErrProc/1(BCMR_bDcComErrDet) -> BCMR_bDcComErrDet/1, [BCMR_bDcComErrDet]
  ComErrProc/2(BCMR_bDcComErrHeal) -> BCMR_bDcComErrHeal/1
  OtherErrProc/1(BCMR_stOtherErr) -> BCMR_stOtherErr/1, [BCMR_stOtherErr]
  DFC_DChrgPosStuckMin/1 -> RelayErrProc/4(DFC_DChrgPosStuckMin)
  DFC_MNegStuckMax/1 -> RelayErrProc/5(DFC_MNegStuckMax)
  DFC_MNegStuckMin/1 -> RelayErrProc/6(DFC_MNegStuckMin)
  DFC_PosStuckMax/1 -> RelayErrProc/7(DFC_PosStuckMax)
  DFC_MPosStuckMin/1 -> RelayErrProc/8(DFC_MPosStuckMin)
  DFC_PrStuckMin/1 -> RelayErrProc/9(DFC_PrStuckMin)
  DFC_DChrgPosStuckMax/1 -> RelayErrProc/3(DFC_DChrgPosStuckMax)
  DFC_DChrgNegStuckMin/1 -> RelayErrProc/2(DFC_DChrgNegStuckMin)
  DFC_DChrgNegStuckMax/1 -> RelayErrProc/1(DFC_DChrgNegStuckMax)
  DFC_SocRngHiMax/1 -> SocErrProc/1(DFC_SocRngHiMax)
  DFC_SocRngHiMin/1 -> SocErrProc/2(DFC_SocRngHiMin)
  DFC_SocRngLoMax/1 -> SocErrProc/3(DFC_SocRngLoMax)
  DFC_SocRngLoMin/1 -> SocErrProc/4(DFC_SocRngLoMin)
  DFC_BattTAlrmMax/1 -> TempErrProc/3(DFC_BattTAlrmMax)
  DFC_BattTFaultMax/1 -> TempErrProc/4(DFC_BattTFaultMax)
  "DFC_BattTWarnMax "/1 -> TempErrProc/5("DFC_BattTWarnMax ")
  DFC_BattTAlrmMin/1 -> TempErrProc/6(DFC_BattTAlrmMin)
  DFC_BattTFaultMin/1 -> TempErrProc/7(DFC_BattTFaultMin)
  DFC_BattTWarnMin/1 -> TempErrProc/8(DFC_BattTWarnMin)
  BSPR_uKl30/1 -> DChrgCnntChk/3(BSPR_uKl30), [BSPR_uKl30]
  [BSPR_uKl30] -> ContErrProc/2(BSPR_uKl30)
  TempErrProc/1(BCMR_bDChrgTempLowErrDet) -> BCMR_bDChrgTempLowErrDet/1
  CurrChk/1(Flg) -> Logical Operator/2
  [COMR_flgRxCCS] -> OverVoltProc/5(COMR_flgRxCCS)
  OverCurrProc/10(BCMR_bDChrgCurrModifyEna) -> BCMR_bDChrgLowTempCurrModifyEna/1
  [BCMR_bDChrgWkup] -> OverCurrProc/8(BCMR_bDChrgWkup)
  [BCMR_stDChrgCnntErr] -> ChrgStopProc/10(BCMR_stChrgCnntErr)
  OverCurrProc/11(BCMR_bDChrgLowTempCurrOvrCnt) -> BCMR_bDChrgLowTempCurrOvrCnt/1  "BCMR_bDChrgLowTempCurrOvrCnt"
  BCMR_flgDChrgStopCActive/1 -> DChrgDFC/2(BCMR_flgDChrgStopCActive)
  Data Type Conversion/1 -> BCMR_stDChrgModeBcl/1  "BCMR_stDChrgModeBcl"
  COMR_flgRxCCS/1 -> OverCurrProc/7(COMR_flgRxCCS), [COMR_flgRxCCS]
  BSPR_uCellVoltMax/1 -> OverCurrProc/9(BSPR_uCellVoltMax), OverVoltProc/1(BSPR_uCellVoltMax)
  OverCurrProc/9(BCMR_stBattDChrgCurrOvrErr) -> [BCMR_stBattDChrgCurrOvrErr], BCMR_stBattDChrgCurrOvrErr/1  "BCMR_stBattDChrgCurrOvrErr"
  OverCurrProc/12(BCMR_bDChrgCutOffVoltOvrCurrDet) -> BCMR_bDChrgCutOffVoltOvrCurrDet/1
  OverCurrProc/13(BCMR_bDChrgCutOffVoltOvrCurrHeal) -> BCMR_bDChrgCutOffVoltOvrCurrHeal/1
  [BCMR_bDChrgFobd] -> DChrgDFC/3(BCMR_bDChrgFobd)
  BCMR_bStakeParaOk/1 -> Terminator/1
  BCMR_flgTxBEM/1 -> DChrgDFC/4(BCMR_flgTxBEM)
  OverVoltProc/4(BCMR_bDChrgOvrSafeCellVoltDet) -> BCMR_bDChrgOvrSafeCellVoltDet/1
  OverVoltProc/5(BCMR_bDChrgOvrSafeCellVoltHeal) -> BCMR_bDChrgOvrSafeCellVoltHeal/1
  ContErrProc/1(BCMR_stDChrgCnntErr) -> [BCMR_stDChrgCnntErr], BCMR_stDChrgCnntErr/1
  ContErrProc/2(BCMR_bChrgCnnttErrHeal) -> BCMR_bChrgCnnttErrHeal/1
  ContErrProc/3(BCMR_bChrgCnnttErrDet) -> BCMR_bChrgCnnttErrDet/1
  ContErrProc/4(BCMR_bDcOutputContErrDet) -> BCMR_bDcOutputContErrDet/1
  ContErrProc/5(BCMR_bDcOutputContErrHeal) -> BCMR_bDcOutputContErrHeal/1
  ContErrProc/6(BCMR_stCC2ChkVoltErr) -> [BCMR_stCC2ChkVoltErr], BCMR_stCC2ChkVoltErr/1
  ContErrProc/7(BCMR_bCC2VolttLowErrDet) -> BCMR_bCC2VolttLowErrDet/1
  ContErrProc/8(BCMR_bCC2VoltLowErrHeal) -> BCMR_bCC2VoltLowErrHeal/1
  ContErrProc/9(BCMR_bCC2VoltHighErrDet) -> BCMR_bCC2VoltHighErrDet/1
  ContErrProc/10(BCMR_bCC2VoltHighErrHeal) -> BCMR_bCC2VoltHighErrHeal/1
  [BCMR_bDChrgWkup] -> DChrgDFC/5(BCMR_bDChrgWkup)
  Logical Operator/1 -> [CurrEna], OverCurrProc/1(CurrEna)
  [CurrEna] -> OverVoltProc/6(CurrEna)
  [BCMR_bDChrgWkup] -> IntetOvrTempCalc/4(BCMR_bDChrgWkup)
  [BCMR_bDChrgWkup] -> TempErrProc/2(BCMR_bDChrgWkup)
  COMR_bChrgStopActive/1 -> ChrgStopProc/16(COMR_bChrgStopActive)
  ChrgStopProc/3(BCMR_bDChrgFltFobd) -> [BCMR_bDChrgFltFobd]
  [BCMR_bDChrgFltFobd] -> DChrgDFC/6(BCMR_bDChrgFltFobd)
  DSMR_stFaultRank/1 -> OtherErrProc/2(DSMR_stFaultRank)
  HVSR_flgHvilFault/1 -> OtherErrProc/3(HVSR_flgHvilFault)
  [BCMR_bDcComErrDet] -> OtherErrProc/4(BCMR_bDcComErrDet)
  [COMR_stPwrUpDwnVcuReq] -> OtherErrProc/5(COMR_stPwrUpDwnVcuReq)
  BSPR_tBattTempMax/1 -> TempErrProc/1(BSPR_tBattTempMax)
  [BCMR_stDChrgMode] -> OtherErrProc/6(BCMR_stDChrgMode)
  COMR_stVcuFalutLvl/1 -> OtherErrProc/1(COMR_stVcuFalutLvl)
  GcRTE_EvccDtc_numb/1 -> Switch2/1
  Constant2/1 -> Switch2/2
  Constant3/1 -> Switch2/3
  Switch2/1 -> EVCC/1(GcRTE_EvccDtc_numb)
  DChrgCnntChk/2(BCMR_bDChrgCnnt) -> BCMR_bDChrgCnnt/1
  DChrgCnntChk/1(BCMR_bDChrgWkup) -> [BCMR_bDChrgWkup], BCMR_bDChrgWkup/1
  BCMR_bDChrgFul/1 -> ChrgStopProc/14(BCMR_bDChrgFul)
  BSER_rSocDspl/1 -> ChrgStopProc/15(BSER_rSocDspl)
  [BCMR_stOtherErr] -> Compare To Constant2/1
  Compare To Constant2/1 -> Switch1/2
  Constant4/1 -> Switch1/1
  BCMR_stDChrgGbFlowTimeout/1 -> Switch1/3
  Switch1/1 -> DChrgDFC/1(BCMR_stDChrgGbFlowTimeout)
  BSPR_uDChrgVolt/1 -> OverVoltProc/2(BSPR_uDChrgVolt)

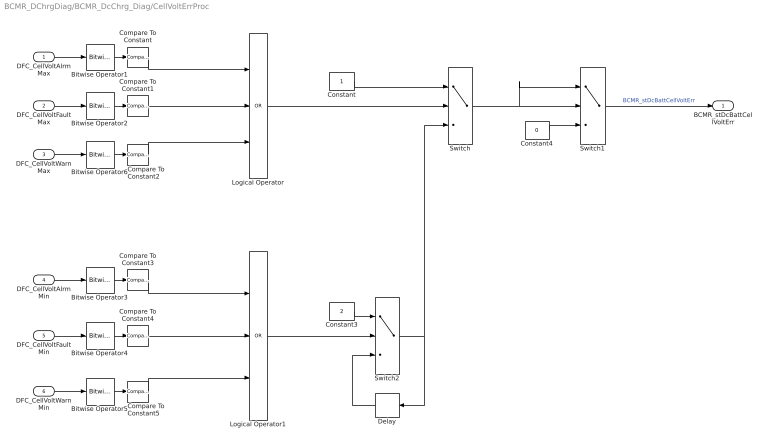
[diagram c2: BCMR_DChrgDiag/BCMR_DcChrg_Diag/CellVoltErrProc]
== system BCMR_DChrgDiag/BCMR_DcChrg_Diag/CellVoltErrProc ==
  DFC_CellVoltAlrmMax : Inport
  DFC_CellVoltFaultMax : Inport  Port=2
  DFC_CellVoltWarnMax : Inport  Port=3
  DFC_CellVoltAlrmMin : Inport  Port=4
  DFC_CellVoltFaultMin : Inport  Port=5
  DFC_CellVoltWarnMin : Inport  Port=6
  Bitwise Operator{1..6} (6 alike) : simulink/Logic and Bit Operations/Bitwise Operator  logicop=AND  UseBitMask=on  BitMask=bin2dec('00011000')  BitMaskRealWorld=Stored Integer
  Compare To Constant{,1..5} (6 alike) : simulink/Logic and Bit Operations/Compare To Constant  relop===  const=24  OutDataTypeStr=boolean
  Constant : Constant  OutDataTypeStr=uint8
  Constant3 : Constant  Value=2  OutDataTypeStr=uint8
  Constant4 : Constant  Value=0  OutDataTypeStr=uint8
  Delay : Delay  DelayLength=1  InitialCondition=0
  Logical Operator : Logic  Operator=OR  Inputs=3  AllPortsSameDT=off  OutDataTypeStr=boolean
  Logical Operator1 : Logic  Operator=OR  Inputs=3  AllPortsSameDT=off  OutDataTypeStr=boolean
  Switch : Switch  Criteria=u2 > Threshold
  Switch1 : Switch  Criteria=u2 > Threshold
  Switch2 : Switch  Criteria=u2 > Threshold
  BCMR_stDcBattCellVoltErr : Outport
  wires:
  Logical Operator/1 -> Switch/2
  Switch/1 -> Switch1/2, Switch1/1
  Constant/1 -> Switch/1
  Constant3/1 -> Switch2/1
  Switch2/1 -> Delay/1, Switch/3
  Switch1/1 -> BCMR_stDcBattCellVoltErr/1  "BCMR_stDcBattCellVoltErr"
  DFC_CellVoltAlrmMax/1 -> Bitwise Operator1/1
  DFC_CellVoltWarnMax/1 -> Bitwise Operator6/1
  DFC_CellVoltFaultMax/1 -> Bitwise Operator2/1
  DFC_CellVoltAlrmMin/1 -> Bitwise Operator3/1
  DFC_CellVoltFaultMin/1 -> Bitwise Operator4/1
  DFC_CellVoltWarnMin/1 -> Bitwise Operator5/1
  Compare To Constant/1 -> Logical Operator/1
  Logical Operator1/1 -> Switch2/2
  Delay/1 -> Switch2/3
  Constant4/1 -> Switch1/3
  Bitwise Operator1/1 -> Compare To Constant/1
  Bitwise Operator2/1 -> Compare To Constant1/1
  Bitwise Operator6/1 -> Compare To Constant2/1
  Compare To Constant2/1 -> Logical Operator/3
  Bitwise Operator3/1 -> Compare To Constant3/1
  Compare To Constant3/1 -> Logical Operator1/1
  Bitwise Operator4/1 -> Compare To Constant4/1
  Compare To Constant4/1 -> Logical Operator1/2
  Bitwise Operator5/1 -> Compare To Constant5/1
  Compare To Constant5/1 -> Logical Operator1/3
  Compare To Constant1/1 -> Logical Operator/2

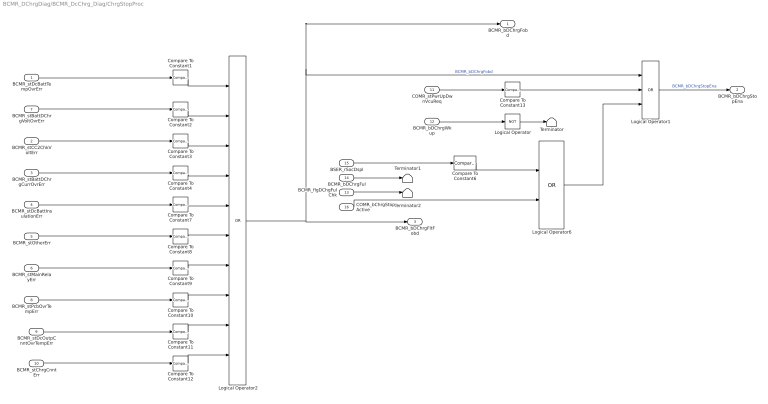
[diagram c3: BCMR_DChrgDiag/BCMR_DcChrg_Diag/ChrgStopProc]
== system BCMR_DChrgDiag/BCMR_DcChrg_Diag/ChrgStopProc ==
  BCMR_stDcBattTempOvrErr : Inport
  BCMR_stCC2ChkVoltErr : Inport  Port=2
  BCMR_stBattDChrgCurrOvrErr : Inport  Port=3
  BCMR_stDcBattInsulationErr : Inport  Port=4
  BCMR_stOtherErr : Inport  Port=5
  BCMR_stMainRelayErr : Inport  Port=6
  BCMR_stBattDChrgVoltOvrErr : Inport  Port=7
  BCMR_stPcbOvrTempErr : Inport  Port=8
  BCMR_stDcOutpCnntOvrTempErr : Inport  Port=9
  BCMR_stChrgCnntErr : Inport  Port=10
  COMR_stPwrUpDwnVcuReq : Inport  Port=11
  BCMR_bDChrgWkup : Inport  Port=12
  BCMR_flgDChgFulChk : Inport  Port=13
  BCMR_bDChrgFul : Inport  Port=14
  BSER_rSocDspl : Inport  Port=15
  COMR_bChrgStopActive : Inport  Port=16
  Compare To Constant{1..4,7..12} (10 alike) : simulink/Logic and Bit Operations/Compare To Constant  relop===  const=1  OutDataTypeStr=boolean
  Compare To Constant13 : simulink/Logic and Bit Operations/Compare To Constant  relop===  const=2  OutDataTypeStr=boolean
  Compare To Constant6 : simulink/Logic and Bit Operations/Compare To Constant  relop=>=  const=100  OutDataTypeStr=boolean
  Logical Operator : Logic  Operator=NOT  AllPortsSameDT=off  OutDataTypeStr=boolean
  Logical Operator1 : Logic  Operator=OR  Inputs=3  AllPortsSameDT=off  OutDataTypeStr=boolean
  Logical Operator2 : Logic  Operator=OR  Inputs=10  AllPortsSameDT=off  OutDataTypeStr=boolean
  Logical Operator6 : Logic  Operator=OR  AllPortsSameDT=off  OutDataTypeStr=boolean
  Terminator : Terminator
  Terminator1 : Terminator
  Terminator2 : Terminator
  BCMR_bDChrgFobd : Outport  OutputWhenDisabled=reset  InitialOutput=[0]
  BCMR_bDChrgStopEna : Outport  Port=2  OutputWhenDisabled=reset  InitialOutput=[0]
  BCMR_bDChrgFltFobd : Outport  Port=3  OutputWhenDisabled=reset  InitialOutput=[0]
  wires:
  BCMR_stDcBattTempOvrErr/1 -> Compare To Constant1/1
  BCMR_stBattDChrgVoltOvrErr/1 -> Compare To Constant2/1
  BCMR_stCC2ChkVoltErr/1 -> Compare To Constant3/1
  BCMR_stBattDChrgCurrOvrErr/1 -> Compare To Constant4/1
  BCMR_stDcBattInsulationErr/1 -> Compare To Constant7/1
  BCMR_stOtherErr/1 -> Compare To Constant8/1
  BCMR_stMainRelayErr/1 -> Compare To Constant9/1
  BCMR_stPcbOvrTempErr/1 -> Compare To Constant10/1
  BCMR_stDcOutpCnntOvrTempErr/1 -> Compare To Constant11/1
  BCMR_stChrgCnntErr/1 -> Compare To Constant12/1
  BCMR_bDChrgWkup/1 -> Logical Operator/1
  COMR_stPwrUpDwnVcuReq/1 -> Compare To Constant13/1
  Compare To Constant13/1 -> Logical Operator1/2
  Logical Operator1/1 -> BCMR_bDChrgStopEna/1  "BCMR_bDChrgStopEna"
  Logical Operator/1 -> Terminator/1
  Logical Operator2/1 -> Logical Operator1/1, BCMR_bDChrgFobd/1, BCMR_bDChrgFltFobd/1  "BCMR_bDChrgFobd"
  Compare To Constant1/1 -> Logical Operator2/1
  Compare To Constant2/1 -> Logical Operator2/2
  Compare To Constant3/1 -> Logical Operator2/3
  Compare To Constant4/1 -> Logical Operator2/4
  Compare To Constant7/1 -> Logical Operator2/5
  Compare To Constant8/1 -> Logical Operator2/6
  Compare To Constant9/1 -> Logical Operator2/7
  Compare To Constant10/1 -> Logical Operator2/8
  Compare To Constant11/1 -> Logical Operator2/9
  Compare To Constant12/1 -> Logical Operator2/10
  BSER_rSocDspl/1 -> Compare To Constant6/1
  Compare To Constant6/1 -> Logical Operator6/1
  Logical Operator6/1 -> Logical Operator1/3
  COMR_bChrgStopActive/1 -> Logical Operator6/2
  BCMR_bDChrgFul/1 -> Terminator1/1
  BCMR_flgDChgFulChk/1 -> Terminator2/1

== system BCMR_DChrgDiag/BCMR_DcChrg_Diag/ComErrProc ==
  COMR_bDcCanBusOff : Inport
  Constant1 : Constant  Value=BCMR_tiDChrgHealDiagDebs_C
  Constant2 : Constant  Value=BCMR_tiDChrgDiagBase_C
  Constant4 : Constant  Value=BCMR_tiDChrgDetDiagDebs_C
  Constant7 : Constant  Value=BCMR_tiDChrgDiagBase_C
  Logical Operator2 : Logic  Operator=NOT  AllPortsSameDT=off  OutDataTypeStr=boolean
  TONV_VariableTimeDebounce : Subsystem  TreatAsAtomicUnit=on  RTWFcnName=TONV_VariableTimeDebounce  RTWFileName=SrvLib
  TONV_VariableTimeDebounce1 : Subsystem  TreatAsAtomicUnit=on  RTWFcnName=TONV_VariableTimeDebounce  RTWFileName=SrvLib
  BCMR_bDcComErrDet : Outport
  BCMR_bDcComErrHeal : Outport  Port=2
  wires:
  COMR_bDcCanBusOff/1 -> TONV_VariableTimeDebounce/1(u), Logical Operator2/1
  TONV_VariableTimeDebounce/1(y) -> BCMR_bDcComErrDet/1  "BCMR_bDcComErrDet"
  TONV_VariableTimeDebounce1/1(y) -> BCMR_bDcComErrHeal/1  "BCMR_bDcComErrHeal"
  Constant7/1 -> TONV_VariableTimeDebounce/3(dT)
  Constant4/1 -> TONV_VariableTimeDebounce/2(T)
  Constant1/1 -> TONV_VariableTimeDebounce1/2(T)
  Logical Operator2/1 -> TONV_VariableTimeDebounce1/1(u)
  Constant2/1 -> TONV_VariableTimeDebounce1/3(dT)

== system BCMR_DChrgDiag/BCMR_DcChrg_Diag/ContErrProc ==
  BSPR_bDCWkUp : Inport
  BSPR_uKl30 : Inport  Port=2
  BSPR_uCC2Volt : Inport  Port=3
  BCMR_stDChrgMode : Inport  Port=4
  APlusDet : Subsystem
  CC2Det : Subsystem
  Compare To Constant : simulink/Logic and Bit Operations/Compare To Constant  relop===  const=2  OutDataTypeStr=boolean
  Compare To Constant1 : simulink/Logic and Bit Operations/Compare To Constant  relop===  const=3  OutDataTypeStr=boolean
  DFC_APlus : Subsystem
  DFC_CC2 : Subsystem
  Logical Operator : Logic  Operator=OR  AllPortsSameDT=off  OutDataTypeStr=boolean
  BCMR_stDChrgCnntErr : Outport  OutputWhenDisabled=reset  InitialOutput=[0]
  BCMR_bChrgCnnttErrHeal : Outport  Port=2  InitialOutput=[0]
  BCMR_bChrgCnnttErrDet : Outport  Port=3  InitialOutput=[0]
  BCMR_bDcOutputContErrDet : Outport  Port=4  InitialOutput=[0]
  BCMR_bDcOutputContErrHeal : Outport  Port=5  InitialOutput=[0]
  BCMR_stCC2ChkVoltErr : Outport  Port=6  OutputWhenDisabled=reset  InitialOutput=[0]
  BCMR_bCC2VolttLowErrDet : Outport  Port=7  InitialOutput=[0]
  BCMR_bCC2VoltLowErrHeal : Outport  Port=8  InitialOutput=[0]
  BCMR_bCC2VoltHighErrDet : Outport  Port=9  InitialOutput=[0]
  BCMR_bCC2VoltHighErrHeal : Outport  Port=10  InitialOutput=[0]
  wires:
  BSPR_bDCWkUp/1 -> APlusDet/1(BSPR_bDCWkUp), CC2Det/Enable
  APlusDet/1(BCMR_bChrgCnnttErrDet) -> DFC_APlus/1(BCMR_bChrgCnnttErrDet), BCMR_bChrgCnnttErrDet/1
  APlusDet/2(BCMR_bChrgCnnttErrHeal) -> DFC_APlus/2(BCMR_bChrgCnnttErrHeal), BCMR_bChrgCnnttErrHeal/1
  BSPR_uKl30/1 -> CC2Det/2(BSPR_uKl30)
  BSPR_uCC2Volt/1 -> CC2Det/1(BSPR_uCC2Volt)
  BCMR_stDChrgMode/1 -> Compare To Constant1/1, Compare To Constant/1
  Compare To Constant/1 -> Logical Operator/1
  Compare To Constant1/1 -> Logical Operator/2
  Logical Operator/1 -> APlusDet/Enable
  CC2Det/2(BCMR_bDcOutputContErrHeal) -> DFC_CC2/2(BCMR_bDcOutputContErrHeal), BCMR_bDcOutputContErrHeal/1  "BCMR_bDcOutputContErrHeal"
  CC2Det/1(BCMR_bDcOutputContErrDet) -> DFC_CC2/1(BCMR_bDcOutputContErrDet), BCMR_bDcOutputContErrDet/1  "BCMR_bDcOutputContErrDet"
  CC2Det/3(BCMR_bCC2VolttLowErrDet) -> DFC_CC2/3(BCMR_bCC2VolttLowErrDet), BCMR_bCC2VolttLowErrDet/1  "BCMR_bCC2VoltLowErrDet"
  CC2Det/4(BCMR_bCC2VoltLowErrHeal) -> DFC_CC2/4(BCMR_bCC2VoltLowErrHeal), BCMR_bCC2VoltLowErrHeal/1  "BCMR_bCC2VoltLowErrHeal"
  CC2Det/5(BCMR_bCC2VoltHighErrDet) -> DFC_CC2/5(BCMR_bCC2VoltHighErrDet), BCMR_bCC2VoltHighErrDet/1  "BCMR_bCC2VoltHighErrDet"
  CC2Det/6(BCMR_bCC2VoltHighErrHeal) -> DFC_CC2/6(BCMR_bCC2VoltHighErrHeal), BCMR_bCC2VoltHighErrHeal/1  "BCMR_bCC2VoltHighErrHeal"
  DFC_CC2/1(BCMR_stCC2ChkVoltErr) -> BCMR_stCC2ChkVoltErr/1
  DFC_APlus/1(BCMR_stDChrgCnntErr) -> BCMR_stDChrgCnntErr/1

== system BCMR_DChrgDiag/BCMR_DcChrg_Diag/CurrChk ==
  Curr : Inport
  Compare To Constant2 : simulink/Logic and Bit Operations/Compare To Constant  relop=<=  const=BCMR_iDChrgCurrDiagLmt_C  OutDataTypeStr=boolean
  Constant3 : Constant  Value=BCMR_tiDChrgDetSec_C
  Constant4 : Constant  Value=BCMR_tiDChrgDiagBase_C
  TONV_TimeDebounce4 : Subsystem  TreatAsAtomicUnit=on
  Flg : Outport
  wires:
  TONV_TimeDebounce4/1(y) -> Flg/1
  Compare To Constant2/1 -> TONV_TimeDebounce4/2(u)
  Curr/1 -> Compare To Constant2/1
  Constant4/1 -> TONV_TimeDebounce4/3(dT)
  Constant3/1 -> TONV_TimeDebounce4/1(T)

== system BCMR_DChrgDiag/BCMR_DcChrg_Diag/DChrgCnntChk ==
  BSPR_bDCWkUp : Inport
  BSPR_uCC2Volt : Inport  Port=2
  BSPR_uKl30 : Inport  Port=3
  Abs : Abs
  Add : Sum  Inputs=+-
  Compare To Constant2 : simulink/Logic and Bit Operations/Compare To Constant  relop===  const=1  OutDataTypeStr=boolean
  Compare To Constant3 : simulink/Logic and Bit Operations/Compare To Constant  relop=<=  const=BCMR_uCC2ChkDiffDet_C  OutDataTypeStr=boolean
  Constant1 : Constant  Value=5.0  OutDataTypeStr=single
  Constant16 : Constant  Value=BCMR_H1U0PlatformSwDiag_C
  Data Type Conversion : DataTypeConversion  OutDataTypeStr=single
  Data Type Conversion1 : DataTypeConversion  OutDataTypeStr=boolean
  Gain : Gain  Gain=0.5
  SIgFil : Subsystem
  Switch1 : Switch  Criteria=u2 ~= 0
  BCMR_bDChrgWkup : Outport
  BCMR_bDChrgCnnt : Outport  Port=2
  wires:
  Compare To Constant2/1 -> BCMR_bDChrgWkup/1  "BCMR_bDChrgWkup"
  Add/1 -> Abs/1
  Abs/1 -> Compare To Constant3/1
  BSPR_bDCWkUp/1 -> Compare To Constant2/1
  BSPR_uCC2Volt/1 -> Add/1
  Constant16/1 -> Switch1/2
  BSPR_uKl30/1 -> Switch1/1
  Constant1/1 -> Switch1/3
  Switch1/1 -> Gain/1
  Gain/1 -> Add/2
  Compare To Constant3/1 -> Data Type Conversion/1
  SIgFil/1(y) -> Data Type Conversion1/1
  Data Type Conversion1/1 -> BCMR_bDChrgCnnt/1  "BCMR_bDChrgCnnt"
  Data Type Conversion/1 -> SIgFil/1(u)
